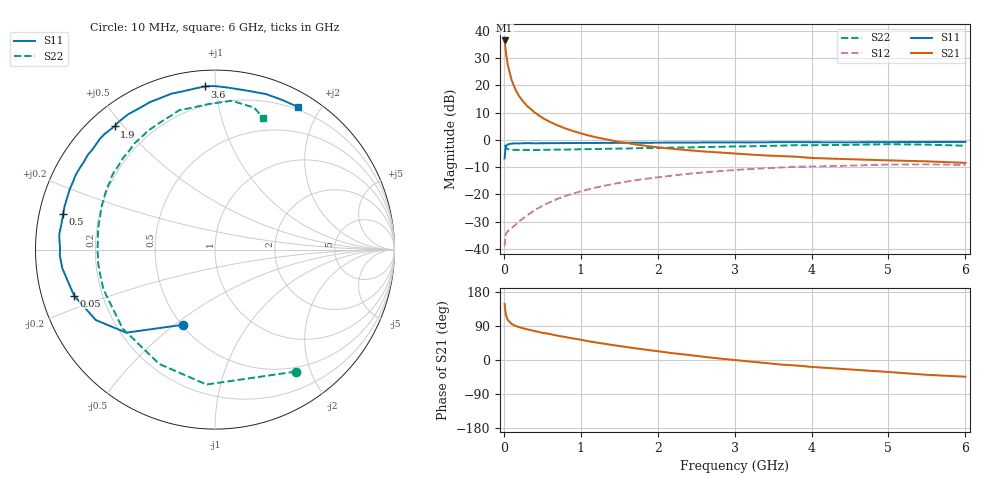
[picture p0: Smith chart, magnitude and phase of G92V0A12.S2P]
! SIEMENS Small Signal Semiconductors
! BFG235
! Si NPN RF Bipolar Junction Transistor in SOT223
! VCE = 2 V  IC = 120 mA
! Common Emitter S-Parameters:  July  1994
# GHz  S  MA  R  50
!  f  S11  S21  S12  S22
! GHz  MAG  ANG  MAG  ANG  MAG  ANG  MAG  ANG
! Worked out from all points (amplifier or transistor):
!   40 points, 10 MHz to 6 GHz, reference 50 ohm
!   highest |S21| = 36.5 dB at 10 MHz (marker M1)
!   |S21| within 3 dB of that: start of sweep to 21.65 MHz
!   unconditionally stable (mu >= 1): 441.2 MHz to 1.586 GHz; 1.841 GHz to 1.911 GHz
!   at 200 MHz: K = 0.81, MSG = 22.9 dB, |S12| = -29.8 dB
!   at 1.5 GHz: K = 1.01, MAG = 6.8 dB, |S12| = -15.8 dB
!   at 6 GHz: K = 0.93, MSG = 0.4 dB, |S12| = -9.2 dB
!   S11 on the Smith chart (normalised r, x): 10 MHz: 0.50, -0.53; 50 MHz: 0.10, -0.16; 500 MHz: 0.07, +0.12; 1.9 GHz: 0.07, +0.47; 3.6 GHz: 0.09, +0.94; 6 GHz: 0.17, +1.73
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0.01  0.4564 -113.3  66.51 148.0  0.0113 58.4  0.815 -56.5
0.02  0.6773 -136.9  49.3 128.3  0.017 43.3  0.7532 -93.6
0.03  0.7714 -149.4  37.33 117.1  0.0192 36.5  0.7089 -116.0
0.05  0.8257 -161.9  24.19 105.9  0.0212 30.9  0.6771 -139.5
0.1  0.8568 -172.9  12.59 95.4  0.0242 35.2  0.66 -160.5
0.15  0.8655 -178.0  8.429 90.1  0.0277 42.0  0.6548 -169.0
0.2  0.8632 179.4  6.299 86.7  0.0322 47.2  0.6555 -173.7
0.25  0.8685 176.5  5.077 83.6  0.0365 51.0  0.6534 -177.0
0.3  0.8716 174.3  4.239 81.2  0.0413 53.7  0.6551 -179.8
0.4  0.8673 170.2  3.193 76.3  0.0516 57.0  0.654 176.3
0.5  0.8691 166.8  2.551 72.0  0.0619 58.5  0.6575 173.0
0.7  0.8733 160.1  1.847 64.1  0.0834 58.7  0.664 167.2
0.9  0.8765 154.7  1.456 56.9  0.104 56.6  0.6695 162.4
1.1  0.8797 148.4  1.207 49.5  0.1244 54.0  0.6782 157.6
1.5  0.8843 138.7  0.918 36.9  0.1631 47.0  0.6949 148.7
1.9  0.8858 129.2  0.761 25.6  0.1983 39.8  0.7106 140.6
2.2  0.8961 122.6  0.686 17.8  0.2231 34.1  0.7239 134.8
3.2  0.8998 101.6  0.541 -4.1  0.2921 14.7  0.7653 116.0
3.6  0.911 93.6  0.506 -12.0  0.3127 6.4  0.7865 107.8
4.5  0.9037 78.5  0.443 -24.9  0.3384 -9.3  0.8122 92.2
5.5  0.9142 65.5  0.405 -39.1  0.3568 -26.9  0.8206 74.6
6  0.919 59.8  0.38 -44.1  0.3468 -33.6  0.7823 70.1
